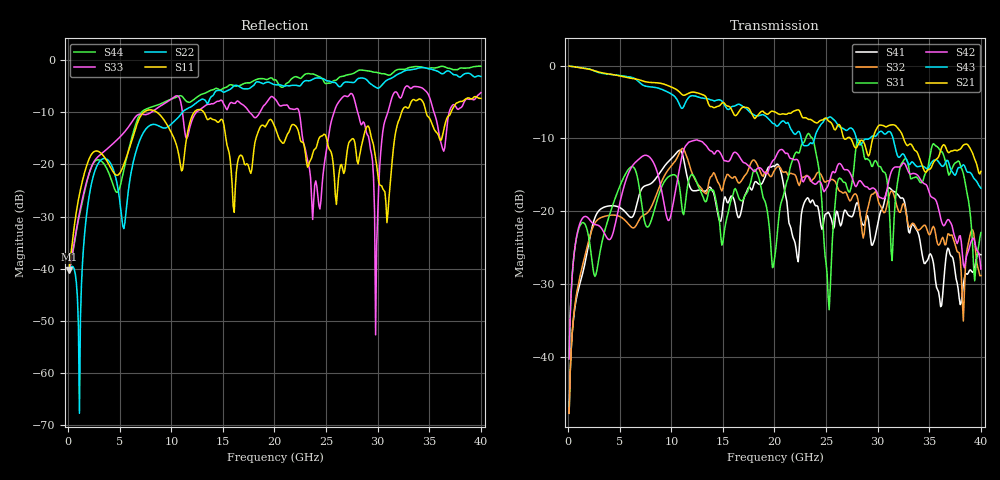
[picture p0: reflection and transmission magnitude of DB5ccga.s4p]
! ADC12DJ3200QML-SP
! 196-pin NWE package
! CCGA Ceramic Package with columns (ceramic column grid array)
! Texas Instruments 4/21/2021
! Single-ended  S-parameters
! PORT#  PORT_NAME  NET_NAME
! PORT1:  DAxN.DIEBUMP DAxN
! PORT2:  DAxN.BGA  DAxN
! PORT3:  DAxP.DIEBUMP DAxP
! PORT4:  DAxP.BGA  DAxP
! Touchstone Ver. 1.0
! Number of ports is 4
# Hz	S	MA	R	50.000000
! SCATTERING PARAMETERS  :
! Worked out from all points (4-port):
!   400 points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, 100 MHz to 40 GHz, reference 50 ohm
!   strongest paths, dB at 100 MHz, 10.1 GHz, 20.1 GHz, 30.1 GHz, 40 GHz:
!     S21: -0.1, -3.0, -6.4, -8.2, -14.5
!     S43: -0.1, -4.0, -8.2, -9.2, -16.8
!     S42: -40.3, -19.6, -12.6, -18.0, -27.9
!     S31: -40.3, -15.0, -25.5, -13.9, -22.9
!     S32: -47.8, -13.6, -14.2, -18.8, -28.9
!     S41: -47.8, -12.6, -13.7, -21.2, -26.0
!   lowest |S11| = -40.2 dB at 100 MHz (marker M1), VSWR 1.02, Z = 51 + j0.169 ohm
!   |S11| at or under -10 dB: start of sweep to 7.354 GHz; 8.6 GHz to 12.23 GHz (3.626 GHz wide, 34.8 % of centre); 13.15 GHz to 32.32 GHz (19.18 GHz wide, 84.4 % of centre)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
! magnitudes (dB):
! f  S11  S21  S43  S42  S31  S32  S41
! 100 MHz  -40.2  -0.1  -0.1  -40.3  -40.3  -47.8  -47.8
! 1.1 GHz  -25.8  -0.3  -0.3  -21.9  -22.2  -29.3  -30.2
! 3.1 GHz  -17.7  -0.9  -1.0  -22.1  -25.6  -20.9  -19.8
! 27.4 GHz  -15.3  -10.0  -8.6  -15.0  -16.9  -18.5  -20.7
! 29.8 GHz  -18.8  -8.9  -9.7  -17.1  -13.1  -17.3  -23.2
! 31.5 GHz  -17.4  -8.1  -10.1  -14.1  -23.7  -17.5  -17.2
! 40 GHz  -7.4  -14.5  -16.8  -27.9  -22.9  -28.9  -26.0
